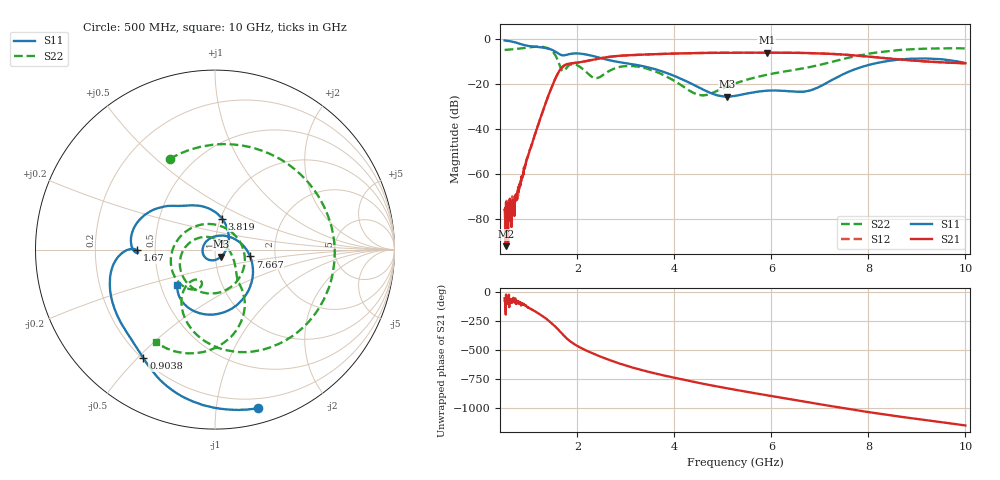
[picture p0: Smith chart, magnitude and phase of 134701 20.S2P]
!  2-Port S-parameters saved by WinCal
! VAR MeasName=S-Parameters (CALIBRATED_DATA) read from VNA (N5242A)
! VAR MeasDate=2013-7-3 16:31:18
! VAR NAME=134701 20
! VAR FILENAME=134701 20.S2P
! VAR DATE=2013-7-3 16:31:18
! VAR PHYS_PORTS=1,2
# Hz S MA R 50
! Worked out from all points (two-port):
!   1601 points, 500 MHz to 10 GHz, reference 50 ohm
!   highest |S21| = -6.19 dB at 5.903 GHz (marker M1); lowest = -92.1 dB at 523.8 MHz (marker M2)
!   |S21| within 3 dB of the highest: 2.349 GHz to 8.642 GHz (6.292 GHz wide, 115 % of centre)
!   lowest |S11| = -25.7 dB at 5.084 GHz (marker M3), VSWR 1.11, Z = 53.4 - j4.16 ohm
!   |S11| at or under -10 dB: 2.764 GHz to 8.369 GHz (5.605 GHz wide, 101 % of centre); 9.821 GHz to end of sweep
!   |S22| runs from -25.2 to -3.5 dB; largest |S21 - S12| = 0.0026
!   S11 on the Smith chart (normalised r, x): 500 MHz: 0.12, -1.30; 903.8 MHz: 0.20, -0.52; 1.67 GHz: 0.39, -0.00; 3.819 GHz: 1.02, +0.36; 7.667 GHz: 1.48, -0.12; 10 GHz: 0.61, -0.26
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5e8  0.9166 -74.8  0.0001588 -57.7  0.0001637 -6.0  0.5645 116.6
5.2375e8  0.9101 -78.1  2.469e-05 163.9  0.00013 -31.8  0.5666 113.2
6.6625e8  0.8578 -97.5  0.0002565 -82.9  0.0002414 -73.7  0.5831 92.2
9.0375e8  0.7245 -123.4  0.001254 -111.3  0.001409 -112.8  0.624 51.6
1.170938e9  0.6592 -144.6  0.01045 -179.5  0.01056 -179.3  0.6685 -5.5
1.384688e9  0.6101 -163.7  0.04852 118.8  0.04861 118.7  0.6217 -62.5
1.539062e9  0.5243 -177.4  0.1256 62.8  0.1252 62.5  0.4419 -109.7
1.669688e9  0.4343 -179.6  0.2233 5.2  0.2228 5.1  0.2088 -125.3
1.865625e9  0.4626 178.7  0.284 -70.5  0.2833 -70.6  0.2683 -128.6
2.085312e9  0.4646 163.3  0.3056 -125.7  0.3048 -125.7  0.2238 171.8
2.530625e9  0.3622 138.1  0.3778 153.5  0.3773 153.5  0.157 0.9
2.904688e9  0.2977 124.7  0.4211 97.8  0.4198 97.7  0.2406 -84.7
3.670625e9  0.2 86.2  0.4573 10.9  0.4567 11.0  0.1765 -179.0
3.819062e9  0.1773 77.1  0.4629 -3.5  0.4627 -3.4  0.1485 165.9
4.525625e9  0.08102 24.2  0.4824 -65.7  0.4826 -65.7  0.05631 66.9
5.08375e9  0.05191 -48.4  0.4881 -109.9  0.4893 -109.9  0.08646 -9.2
5.25e9  0.0538 -71.7  0.4887 -122.5  0.4895 -122.5  0.1014 -19.7
5.903125e9  0.07029 -141.0  0.4901 -169.7  0.4897 -169.9  0.1575 -42.8
6.835312e9  0.07324 91.8  0.479 124.5  0.4789 124.5  0.2403 -54.9
7.666562e9  0.1992 -11.0  0.4294 67.0  0.4303 66.9  0.3948 -66.3
8.420625e9  0.323 -63.8  0.3645 19.5  0.3645 19.3  0.5338 -87.0
1e10  0.2887 -136.6  0.2852 -69.5  0.2848 -69.8  0.6115 -122.6
